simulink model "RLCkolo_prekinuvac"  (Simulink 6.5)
settings: Solver=ode23t  StartTime=0.0  StopTime=1  RelTol=1e-6
undefined symbols (not defined in the file or in its folder): blocks, Continuous, powergui, ZData
libraries: powerlib x7

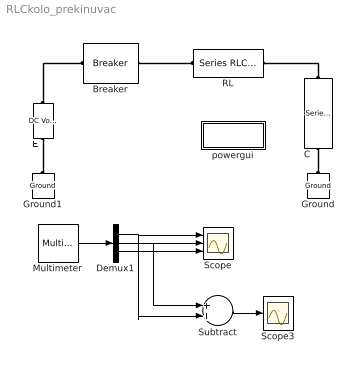
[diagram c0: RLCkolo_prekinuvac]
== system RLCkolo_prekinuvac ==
  Breaker : powerlib/Elements/Breaker  DialogController=PMDialogs.PMDefaultMaskDlg  SystemSampleTime=-1  BreakerResistance=0.01  InitialState=1  SnubberResistance=1e6  SnubberCapacitance=inf  SwitchingTimes=[ 0.3 0.4 ]  External=off  Measurements=None  MoreParameters=off  NoBreakLoop=off
  C : powerlib/Elements/Series RLC Branch  Orientation=down  DialogController=PMDialogs.PMDefaultMaskDlg  PhysicalDomain=powersysdomain  SubClassName=unknown  LeftPortType=p1  RightPortType=p1  LConnTagsString=__new0  RConnTagsString=__new0  BranchType=C  Resistance=1  Inductance=1e-3  SetiL0=off  InitialCurrent=0  Capacitance=100e-6  Setx0=on  InitialVoltage=0  Measurements=Branch voltage and current
  Demux1 : Demux  Outputs=3
  E : powerlib/Electrical Sources/DC Voltage Source  Orientation=up  DialogController=PMDialogs.PMDefaultMaskDlg  SystemSampleTime=-1  Amplitude=12  Measurements=None
  Ground : powerlib/Elements/Ground  Orientation=down  DialogController=PMDialogs.PMDefaultMaskDlg  PhysicalDomain=powersysdomain  SubClassName=unknown  LeftPortType=p1  RightPortType=p1  LConnTagsString=a
  Ground1 : powerlib/Elements/Ground  Orientation=down  DialogController=PMDialogs.PMDefaultMaskDlg  PhysicalDomain=powersysdomain  SubClassName=unknown  LeftPortType=p1  RightPortType=p1  LConnTagsString=a
  Multimeter : powerlib/Measurements/Multimeter  SystemSampleTime=-1  PhasorSimulation=off  OutputType=Complex  sel=[1 2 4]  L=4  Gain=[1 1 1]  yselected={'Ub: C','Ub: RL','Ib: RL'};  PSBOutputType=1  PSBequivalent=0  AxesSetting=[0,0.1,-100,100]  Display=0  SavedBlockNames=-11
  RL : powerlib/Elements/Series RLC Branch  DialogController=PMDialogs.PMDefaultMaskDlg  PhysicalDomain=powersysdomain  SubClassName=unknown  LeftPortType=p1  RightPortType=p1  LConnTagsString=__new0  RConnTagsString=__new0  BranchType=RL  Resistance=3.6  Inductance=0.57  SetiL0=on  InitialCurrent=0  Capacitance=100e-6  Setx0=on  InitialVoltage=0  Measurements=Branch voltage and current
  Scope : Scope  NumInputPorts=3
  Scope3 : Scope
  Subtract : Sum  OutScaling=2^-10
  powergui : Subsystem  AncestorBlock=powerlib/powergui  InitFcn=powergui( 'InitFcn_Callback' , gcb , 0 , [ ] );  mask(PSB option menu block){SimulationMode=Continuous, SampleTime=50e-6, echomessages=off, RestoreLinks=warning, x0status=blocks, Frange=[0:2:500], Ylog=off, Xlog=on, ShowGrid=off, save=off, variable=ZData, structure=, ZoomFFT=on, StartTime=0.0, cycles=1, DisplayStyle=1, fundamental=60, FreqAxis=off, MaxFrequency=1000, frequencyindice=0, frequencyindicesteady=1, RmsSteady=1, display=off, Ts=0, frequency=60, methode=off, HookPort=off, Interpol=off}
      mask prompts: SimulationMode "Simulation mode"; SampleTime "Sample time Ts (when simulation mode is Discrete) (s)"; echomessages "Echo  Messages"; RestoreLinks "Restore disabled links"; x0status "Initial electrical states status"; Frange "Impedance tool: Frequency Range"; Ylog "Impedance tool: Log impedance"; Xlog "Impedance tool: log Frequency"; ShowGrid "Impedance tool: grid"; save "Impedance tool: Save Data To Workspace"; variable "Impedance tool: Variable Name"; structure "Structure Name (PSBFFTSCOPE)"; ZoomFFT "ZoomFFT (PSBFFTSCOPE)"; StartTime "Start Time (PSBFFTSCOPE)"; cycles "Cycles (PSBFFTSCOPE)"; DisplayStyle "Display style (PSBFFTSCOPE)"; fundamental "Fundamental (PSBFFTSCOPE)"; FreqAxis "Frequency Axis (PSBFFTSCOPE)"; MaxFrequency "Max Frequency (PSBFFTSCOPE)"; frequencyindice "Load flow frequency (Hz)"; frequencyindicesteady "Frequency indice (STEADYSTATE)"; RmsSteady "RMS display (STEADYSTATE)"; display "Display Results"; Ts "OBSOLETE 1"; frequency "Phasor frequency (Hz)"; methode "Phasor simulation"; HookPort "Hook port"; Interpol "Interpolate"
      mask init:
      | powerlibroot = which('powersysdomain');
      | PSBroot = powerlibroot(1:end-16);
      | %
      | switch SimulationMode
      | 	case 1
      | 		message=sprintf('Continuous');
      | 	case 2
      |         SampleTimeeval=evalin('base',SampleTime,'NaN');
      |         if isnan(SampleTimeeval)
      |             message=sprintf('Warning !!,\nUndefined sample time');
      |         else
      |             message=sprintf('Discrete,\nTs = %.4g s.',SampleTimeeval);
      |         end
      | 	case 3
      | 		message=sprintf('Phasors');
      | end
      | if strcmp(bdroot,'powerlib')
      |   message='powergui';
      | end
      | power_initmask();
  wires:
  Multimeter/1 -> Demux1/1
  Demux1/1 -> Scope/1, Subtract/2
  Demux1/2 -> Scope/2, Subtract/1
  Demux1/3 -> Scope/3
  Subtract/1 -> Scope3/1
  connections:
  Ground/LConn1 -- C/RConn1
  C/LConn1 -- RL/RConn1
  Ground1/LConn1 -- E/LConn1
  Breaker/RConn1 -- RL/LConn1
  E/RConn1 -- Breaker/LConn1

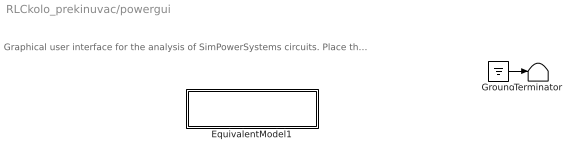
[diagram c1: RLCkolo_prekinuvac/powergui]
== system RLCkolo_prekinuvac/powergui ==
  note: Graphical user interface for the analysis of SimPowerSystems circuits. Place the Powergui block in the top-level of your model and double-click on it to open the GUI.
  EquivalentModel1 : Subsystem
  Ground : Ground
  Terminator : Terminator
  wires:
  Ground/1 -> Terminator/1

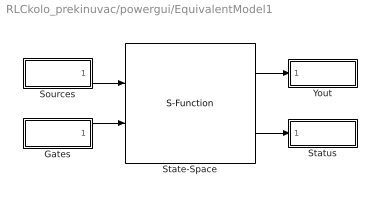
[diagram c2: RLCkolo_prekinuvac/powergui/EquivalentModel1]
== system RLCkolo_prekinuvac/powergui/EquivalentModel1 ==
  Gates : Subsystem
  Sources : Subsystem
  State-Space : S-Function  FunctionName=sfun_spssw_contc  Parameters=A, B, C, D, x0, SwitchResistance ,SwitchType, SwitchGateInitialValue, OutputsToResetToZero
  Status : Subsystem
  Yout : Subsystem
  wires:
  Gates/1(gates) -> State-Space/2
  Sources/1(u) -> State-Space/1
  State-Space/2 -> Status/1(status)
  State-Space/1 -> Yout/1(v,i)

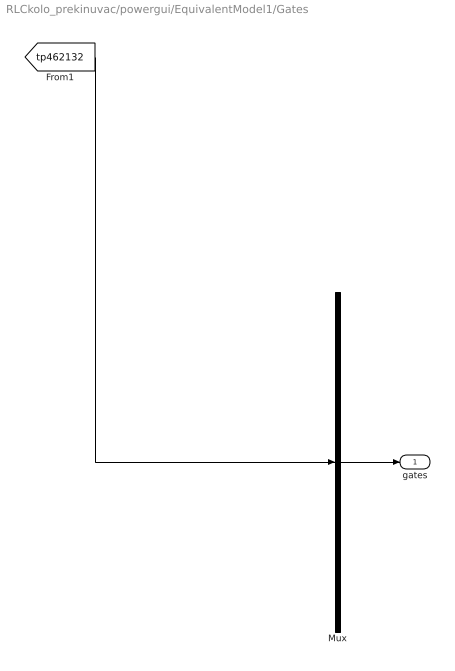
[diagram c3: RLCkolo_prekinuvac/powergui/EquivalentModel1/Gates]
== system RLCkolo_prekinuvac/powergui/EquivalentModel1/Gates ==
  Mux : Mux  Inputs=1
  gates : Outport
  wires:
  Mux/1 -> gates/1
  [tp462132] -> Mux/1

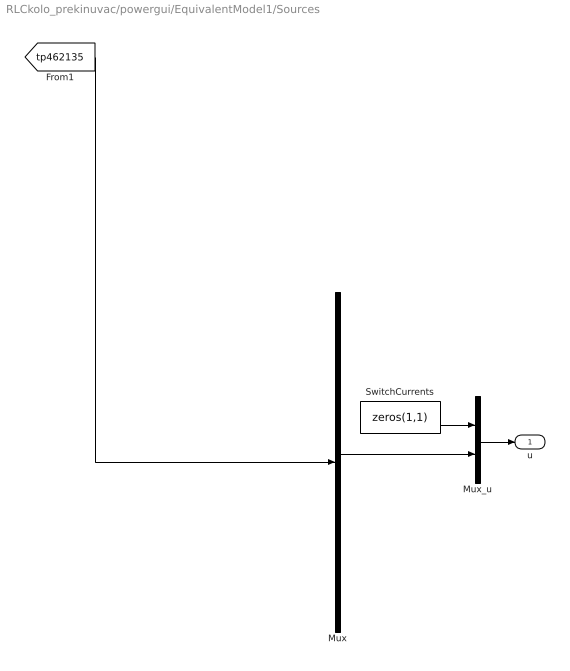
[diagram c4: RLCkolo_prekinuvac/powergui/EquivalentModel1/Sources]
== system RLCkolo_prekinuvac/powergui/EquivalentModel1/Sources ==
  Mux : Mux  Inputs=1
  Mux_u : Mux  Inputs=[1 1]
  SwitchCurrents : Constant  Value=zeros(1,1)  OutDataType=sfix(16)  ConRadixGroup=Use specified scaling  OutScaling=2^0  SampleTime=inf  FramePeriod=inf
  u : Outport
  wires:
  Mux/1 -> Mux_u/2
  SwitchCurrents/1 -> Mux_u/1
  Mux_u/1 -> u/1
  [tp462135] -> Mux/1

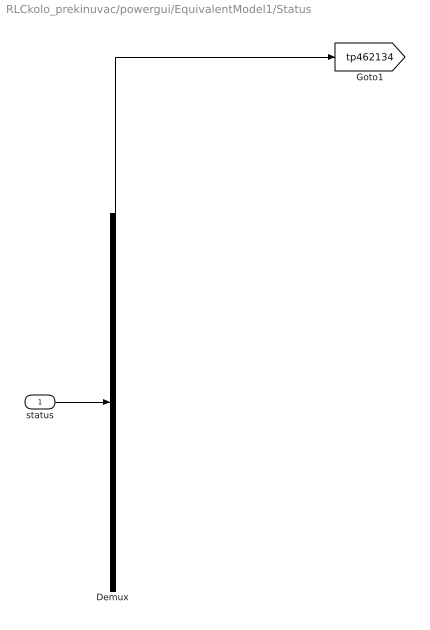
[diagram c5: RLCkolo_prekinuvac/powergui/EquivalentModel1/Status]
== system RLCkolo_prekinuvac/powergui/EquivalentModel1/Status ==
  status : Inport
  Demux : Demux  Outputs=1
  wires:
  status/1 -> Demux/1
  Demux/1 -> [tp462134]

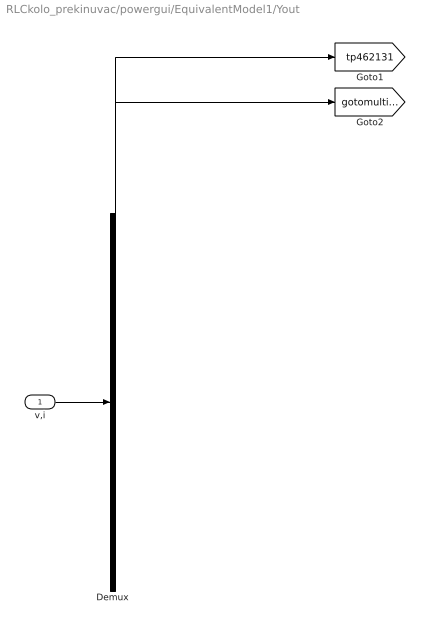
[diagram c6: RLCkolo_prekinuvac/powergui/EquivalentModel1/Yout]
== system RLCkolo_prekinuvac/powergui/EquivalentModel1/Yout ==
  v,i : Inport
  Demux : Demux  Outputs=[1 4]
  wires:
  v,i/1 -> Demux/1
  Demux/1 -> [tp462131]
  Demux/2 -> [gotomultimeterPSB]
